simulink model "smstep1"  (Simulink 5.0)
settings: Solver=ode45  StartTime=0.0  StopTime=8  MaxStep=0.03  RelTol=1e-2

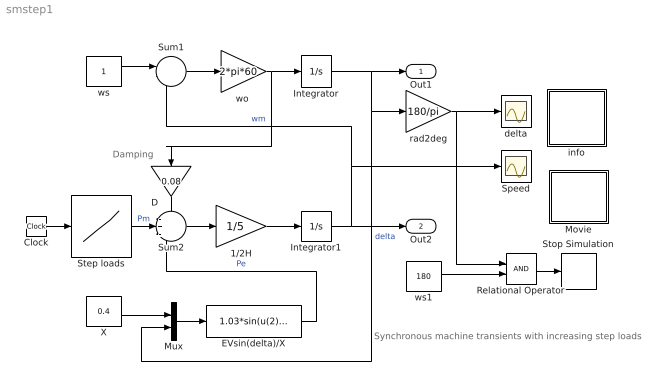
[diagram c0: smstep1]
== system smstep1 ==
  note: Damping
  note: Synchronous machine transients with increasing step loads
  1/2H : Gain  Gain=1/5
  Clock : Clock
  D : Gain  Orientation=down  Gain=0.08
  EVsin(delta)/X : Fcn  Expr=1.03*sin(u(2))/u(1)
  Integrator : Integrator
  Integrator1 : Integrator  InitialCondition=1
  Movie : Subsystem
  Mux : Mux  Inputs=2
  Relational Operator : RelationalOperator
  Speed : Scope
  Step loads : Lookup  InputValues=[0 1 1 3 3 6 6 20]  OutputValues="[0 0 1 1 2.3 2.3   2.6 2.6]"  ShowAdditionalParam=on
  Stop Simulation : Stop
  Sum1 : Sum  Inputs=|-+
  Sum2 : Sum  Inputs=-+-
  X : Constant  Value=0.4
  delta : Scope
  info : Subsystem
  rad2deg : Gain  Gain=180/pi
  "wo " : Gain  Gain=2*pi*60
  ws : Constant
  ws1 : Constant  Value=180
  Out1 : Outport
  Out2 : Outport  Port=2
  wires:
  ws/1 -> Sum1/1
  Integrator/1 -> Mux/2, rad2deg/1, Out1/1  "delta"
  Sum1/1 -> "wo "/1
  Mux/1 -> EVsin(delta)/X/1
  Sum2/1 -> 1/2H/1
  1/2H/1 -> Integrator1/1
  Integrator1/1 -> Sum1/2, Speed/1, Out2/1  "wm"
  Step loads/1 -> Sum2/2  "Pm"
  D/1 -> Sum2/1
  "wo "/1 -> Integrator/1, D/1
  EVsin(delta)/X/1 -> Sum2/3  "Pe"
  X/1 -> Mux/1
  Clock/1 -> Step loads/1
  rad2deg/1 -> delta/1, Relational Operator/1
  ws1/1 -> Relational Operator/2
  Relational Operator/1 -> Stop Simulation/1

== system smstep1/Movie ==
  note: This demo simulates the transient response of a synchronous machine when a series of step loads is applied.
  note: First start the simulation, then double click the block to proceed with the animation procedure.

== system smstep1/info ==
  note: First start the simulation, then double click the block to proceed with the animation procedure.
